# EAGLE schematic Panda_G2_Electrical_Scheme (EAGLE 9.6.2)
AUTHOR: Andrea Maroso; TITLE: Electrical Scheme

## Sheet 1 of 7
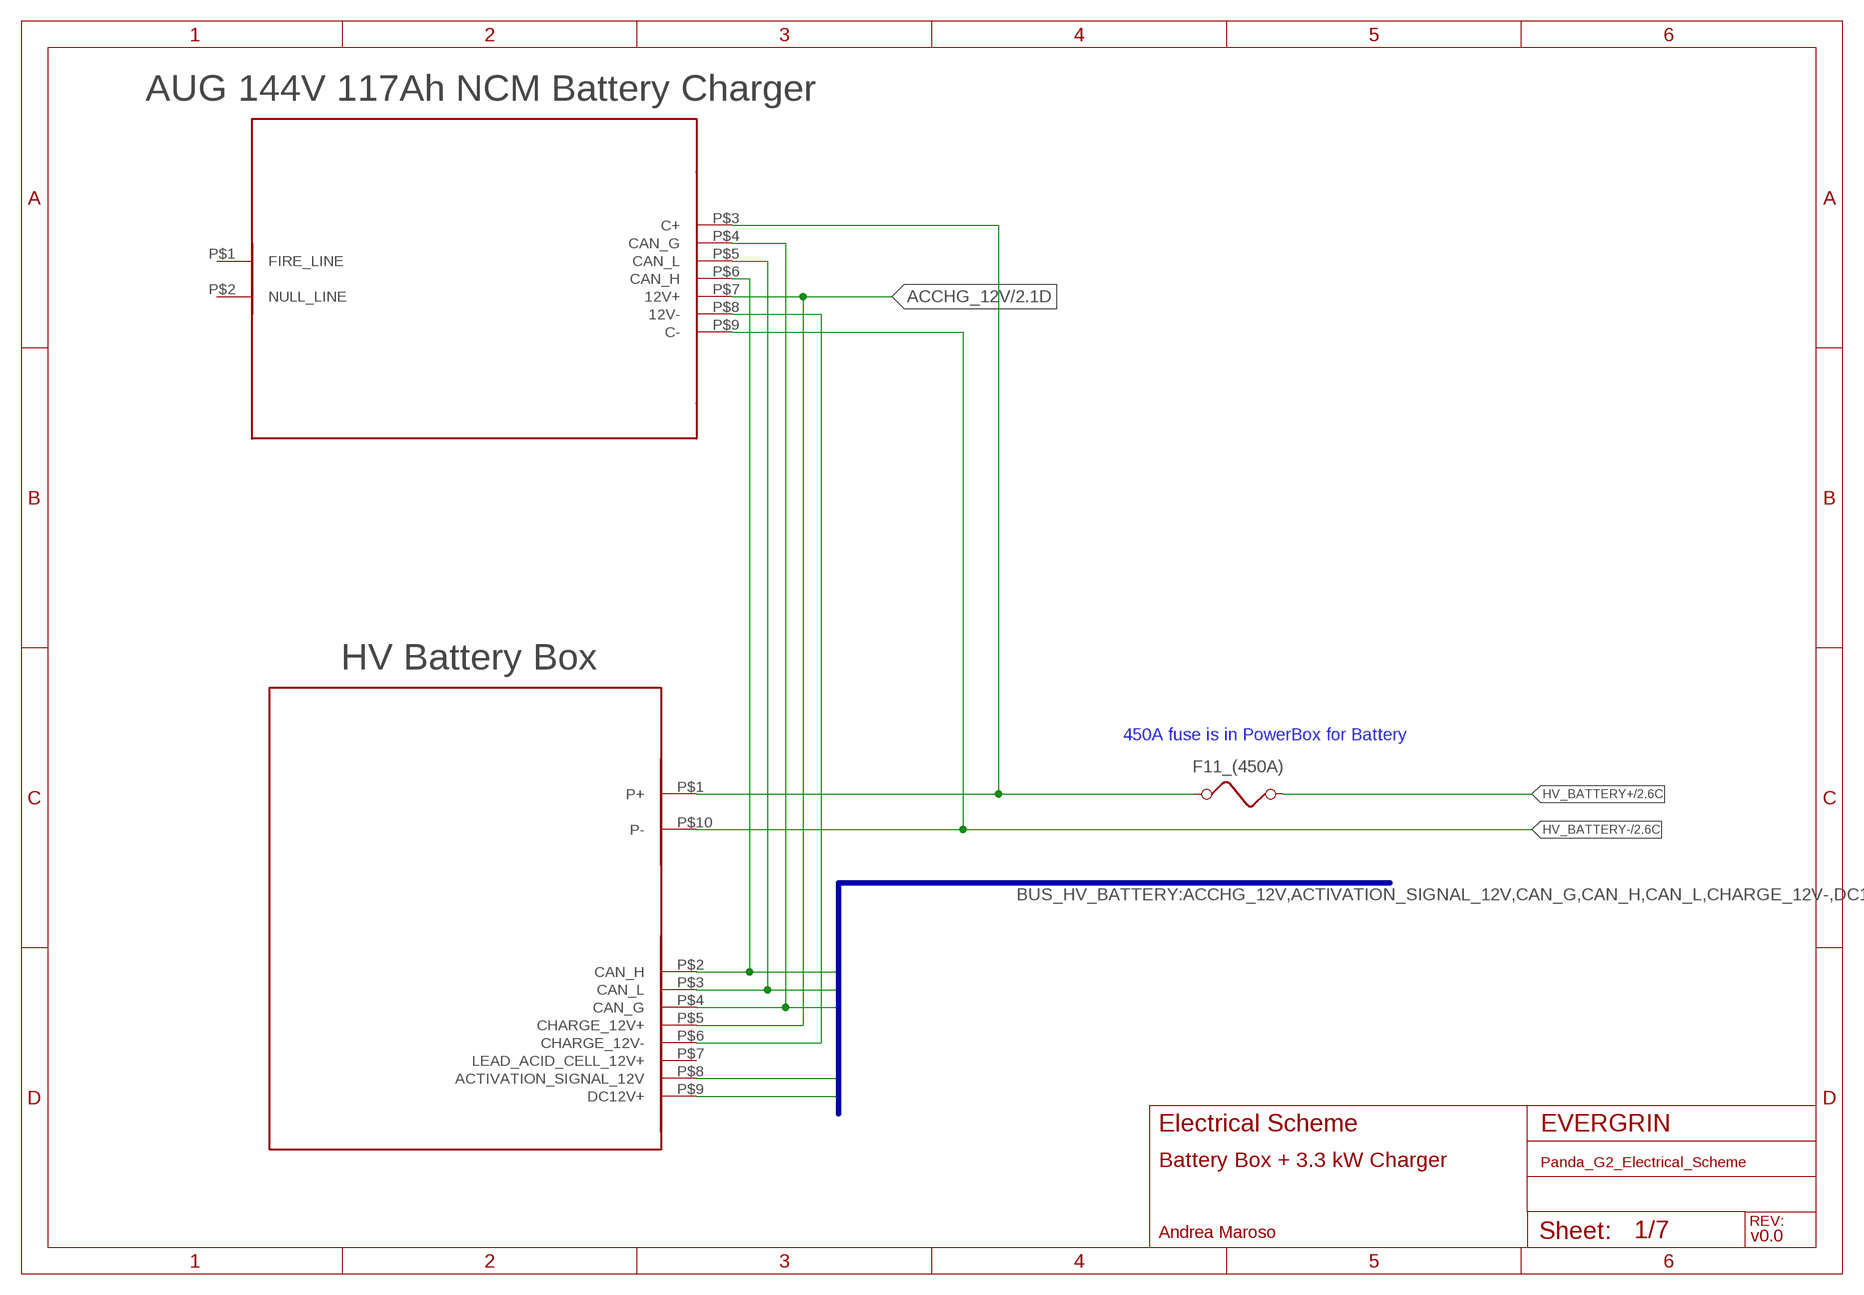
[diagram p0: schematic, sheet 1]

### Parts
F11_(450A)  FUSE  [FUSE]
U$1  HV_BATTERY_BOX  [HV_BATTERY_BOX]
U$2  1.8KW_BATTERY_CHARGER  [1.8KW_BATTERY_CHARGER]

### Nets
ACCHG_12V: U$1.P$5(CHARGE_12V+) U$2.P$7(12V+) ; also sheet 2,6
ACTIVATION_SIGNAL_12V: U$1.P$8(ACTIVATION_SIGNAL_12V) ; also sheet 6
CAN_G: U$1.P$4(CAN_G) U$2.P$4(CAN_G) ; also sheet 6
CAN_H: U$1.P$2(CAN_H) U$2.P$6(CAN_H) ; also sheet 2,6
CAN_L: U$1.P$3(CAN_L) U$2.P$5(CAN_L) ; also sheet 2,6
DC12V+: U$1.P$9(DC12V+) ; also sheet 6
HV_BATTERY+: F11_(450A).1 U$1.P$1(P+) U$2.P$3(C+) ; also sheet 2,4
HV_BATTERY+/2.6C: F11_(450A).2
HV_BATTERY-: U$1.P$10(P-) U$2.P$9(C-) ; also sheet 2,4
N$28: U$1.P$6(CHARGE_12V-) U$2.P$8(12V-)
Unconnected: U$1.P$7(LEAD_ACID_CELL_12V+) U$2.P$1(FIRE_LINE) U$2.P$2(NULL_LINE)

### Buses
BUS_HV_BATTERY:ACCHG_12V,ACTIVATION_SIGNAL_12V,CAN_G,CAN_H,CAN_L,CHARGE_12V-,DC12V+

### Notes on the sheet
- 450A fuse is in PowerBox for Battery
- Battery Box + 3.3 kW Charger
- v0.0

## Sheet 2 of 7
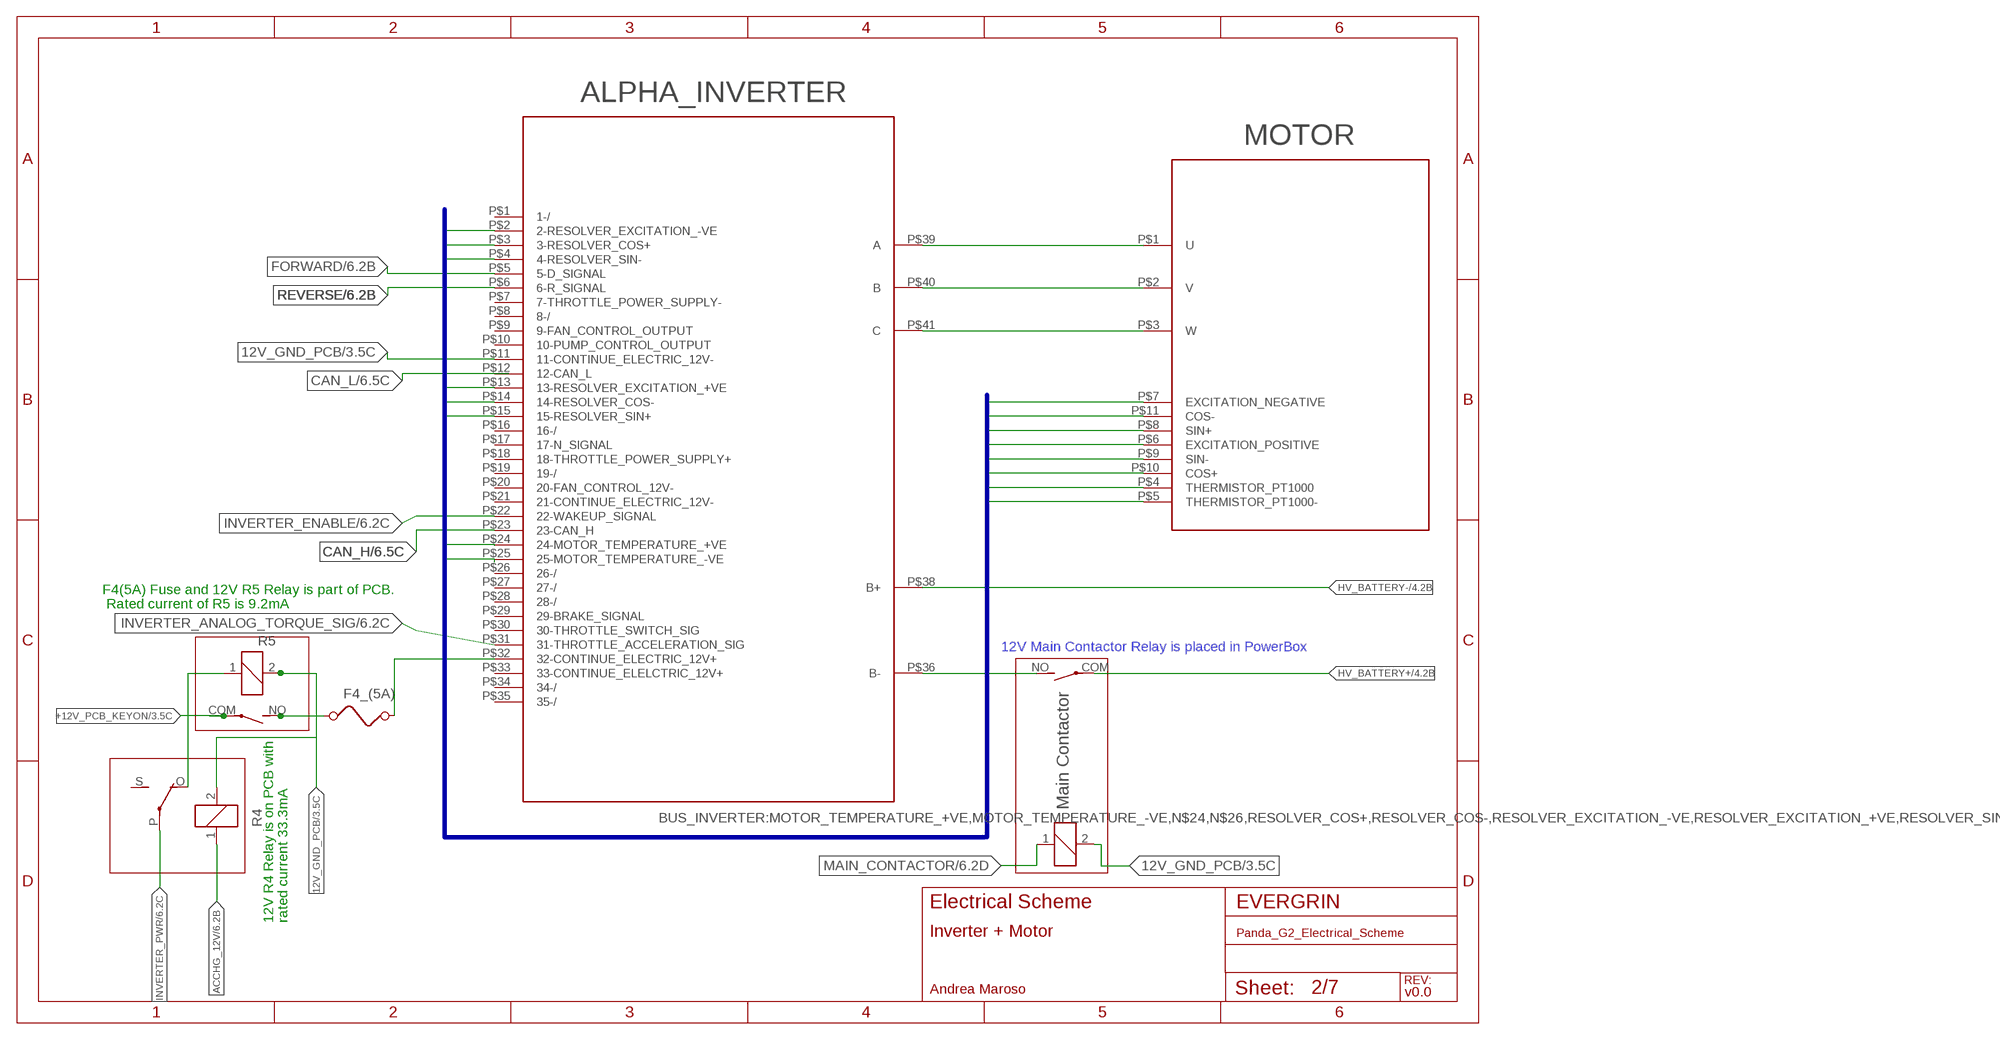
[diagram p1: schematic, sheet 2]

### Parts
F4_(5A)  FUSE  [FUSE]
K1  G5L  [G5LE]
MAIN_CONTACTOR  APF30212A  [APF30212A]
R5  APF30212A  [APF30212A]
U$3  INVERTER  [INVERTER]
U$4  MOTOR  [MOTOR]

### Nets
12V_GND_PCB: K1.2 MAIN_CONTACTOR.2 R5.2 U$3.P$11(11-CONTINUE_ELECTRIC_12V-) ; also sheet 3,4,5,6,7
+12V_PCB_KEYON: R5.COM(2:P) ; also sheet 3,5,7
ACCHG_12V: K1.1 ; also sheet 1,6
CAN_H: U$3.P$23(23-CAN_H) ; also sheet 1,6
CAN_L: U$3.P$12(12-CAN_L) ; also sheet 1,6
FORWARD: U$3.P$5(5-D_SIGNAL) ; also sheet 6
HV_BATTERY+: MAIN_CONTACTOR.COM(2:P) ; also sheet 1,4
HV_BATTERY-: U$3.P$38(B+) ; also sheet 1,4
INVERTER_ANALOG_TORQUE_SIG: U$3.P$31(31-THROTTLE_ACCELERATION_SIG) ; also sheet 6
INVERTER_ENABLE: U$3.P$22(22-WAKEUP_SIGNAL) ; also sheet 6
INVERTER_PWR: K1.P(2:P) ; also sheet 6
MAIN_CONTACTOR: MAIN_CONTACTOR.1 ; also sheet 6
N$1: F4_(5A).2 U$3.P$32(32-CONTINUE_ELECTRIC_12V+)
N$2: U$3.P$39(A) U$4.P$1(U)
N$3: U$3.P$40(B) U$4.P$2(V)
N$4: U$3.P$41(C) U$4.P$3(W)
N$5: MAIN_CONTACTOR.NO(2:S) U$3.P$36(B-)
N$23: F4_(5A).1 R5.NO(2:S)
N$24: U$3.P$24(24-MOTOR_TEMPERATURE_+VE) U$4.P$4(THERMISTOR_PT1000)
N$25: K1.O(2:O) R5.1
N$26: U$3.P$25(25-MOTOR_TEMPERATURE_-VE) U$4.P$5(THERMISTOR_PT1000-)
RESOLVER_COS+: U$3.P$3(3-RESOLVER_COS+) U$4.P$10(COS+)
RESOLVER_COS-: U$3.P$14(14-RESOLVER_COS-) U$4.P$11(COS-)
RESOLVER_EXCITATION_+VE: U$3.P$13(13-RESOLVER_EXCITATION_+VE) U$4.P$6(EXCITATION_POSITIVE)
RESOLVER_EXCITATION_-VE: U$3.P$2(2-RESOLVER_EXCITATION_-VE) U$4.P$7(EXCITATION_NEGATIVE)
RESOLVER_SIN+: U$3.P$15(15-RESOLVER_SIN+) U$4.P$8(SIN+)
RESOLVER_SIN-: U$3.P$4(4-RESOLVER_SIN-) U$4.P$9(SIN-)
REVERSE: U$3.P$6(6-R_SIGNAL) ; also sheet 6
Unconnected: K1.S(2:S) U$3.P$1(1-/) U$3.P$7(7-THROTTLE_POWER_SUPPLY-) U$3.P$8(8-/) U$3.P$9(9-FAN_CONTROL_OUTPUT) U$3.P$10(10-PUMP_CONTROL_OUTPUT) U$3.P$16(16-/) U$3.P$17(17-N_SIGNAL) U$3.P$18(18-THROTTLE_POWER_SUPPLY+) U$3.P$19(19-/) U$3.P$20(20-FAN_CONTROL_12V-) U$3.P$21(21-CONTINUE_ELECTRIC_12V-) U$3.P$26(26-/) U$3.P$27(27-/) U$3.P$28(28-/) U$3.P$29(29-BRAKE_SIGNAL) U$3.P$30(30-THROTTLE_SWITCH_SIG) U$3.P$33(33-CONTINUE_ELELCTRIC_12V+) U$3.P$34(34-/) U$3.P$35(35-/)

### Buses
BUS_INVERTER:MOTOR_TEMPERATURE_+VE,MOTOR_TEMPERATURE_-VE,N$24,N$26,RESOLVER_COS+,RESOLVER_COS-,RESOLVER_EXCITATION_-VE,RESOLVER_EXCITATION_+VE,RESOLVER_SIN-,RESOLVER_SIN+

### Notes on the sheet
- F4(5A) Fuse and 12V R5 Relay is part of PCB.
- Rated current of R5 is 9.2mA
- 12V Main Contactor Relay is placed in PowerBox
- Main Contactor
- R4
- 12V R4 Relay is on PCB with | rated current 33.3mA
- Inverter + Motor
- v0.0

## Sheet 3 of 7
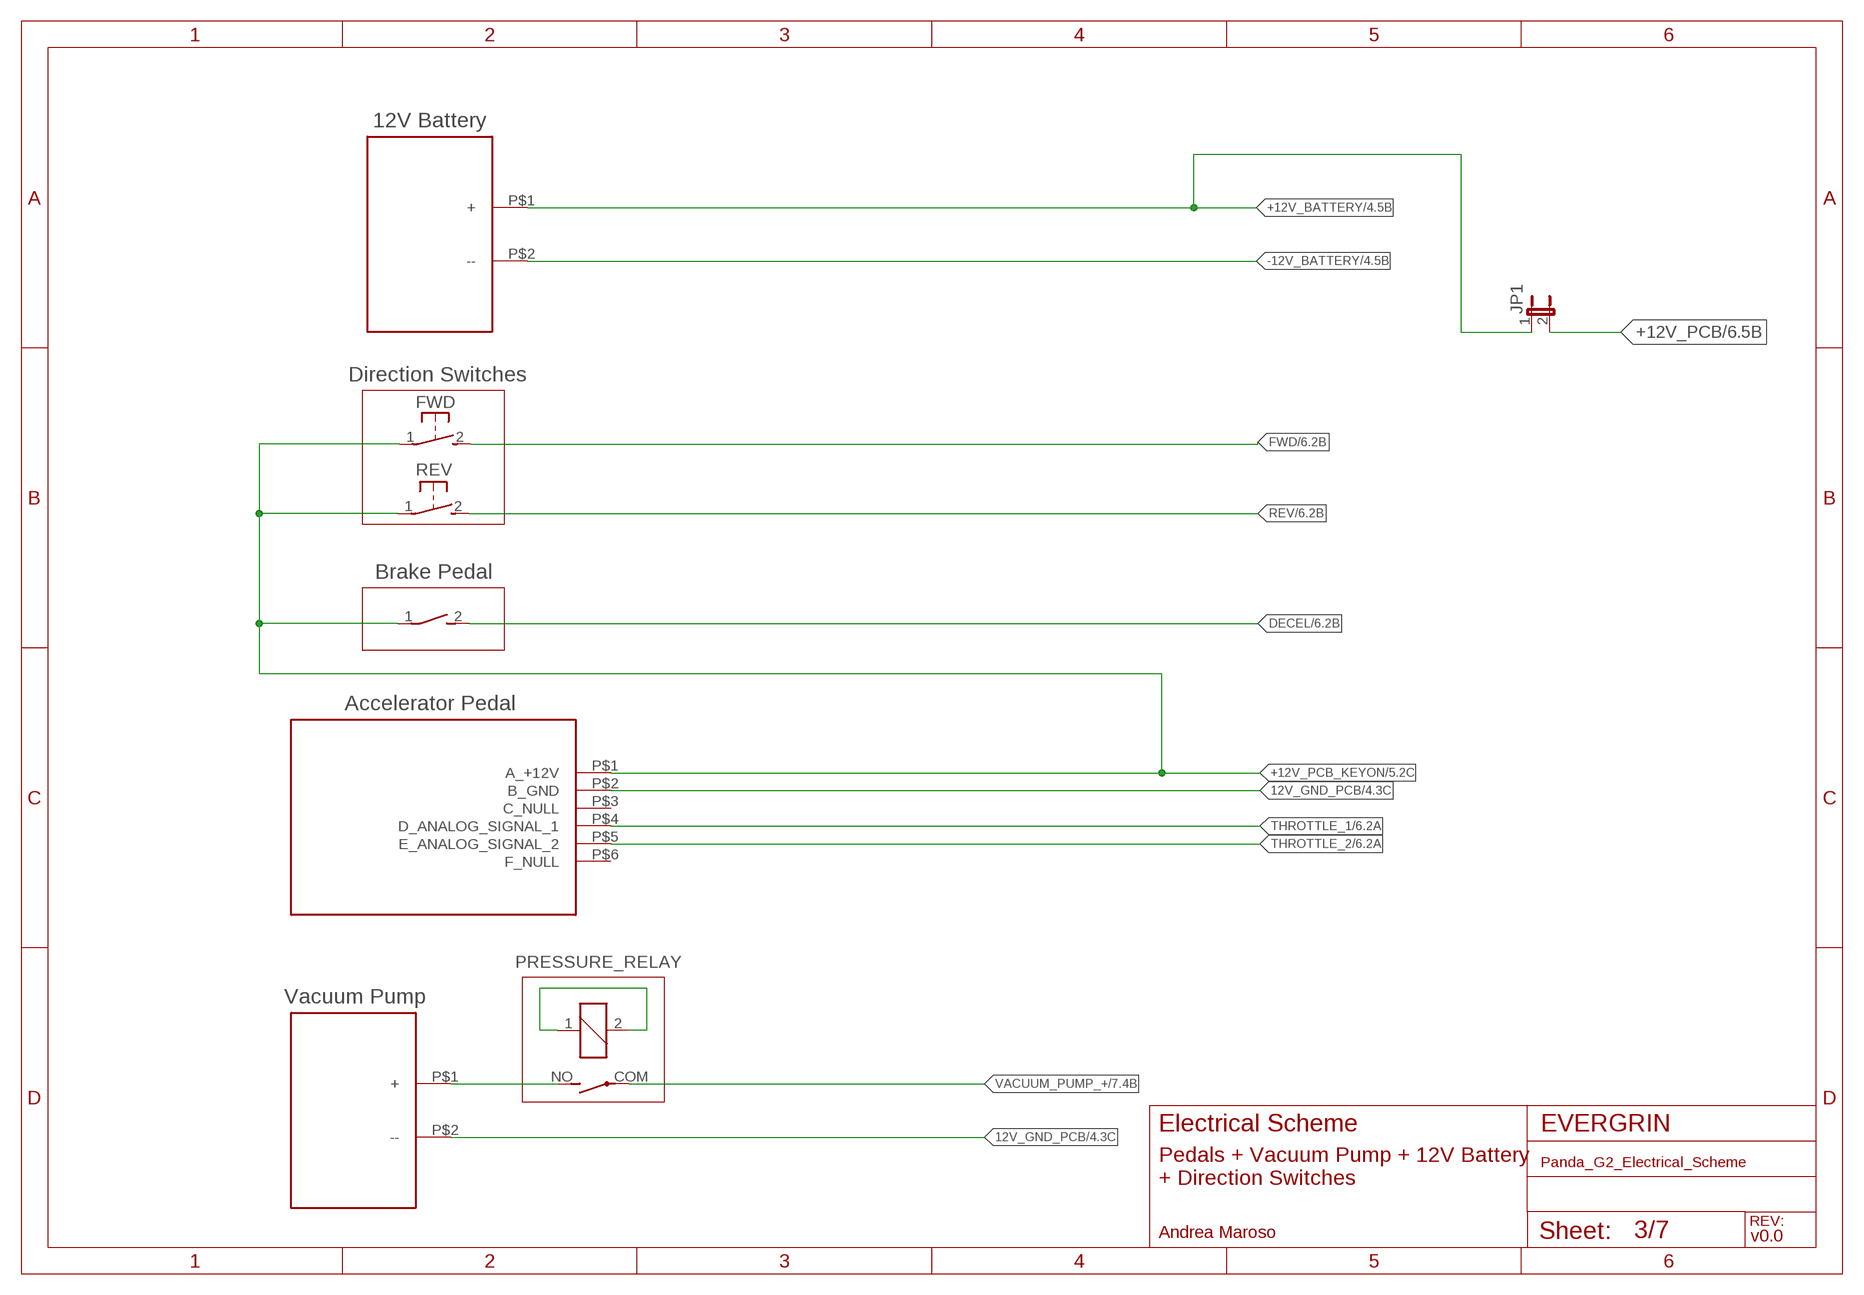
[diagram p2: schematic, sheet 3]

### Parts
JP1  JP1E  [JP1]
PRESSURE_RELAY  APF30212A  [APF30212A]
S1  31-XX  [B3F-31XX]
S2  31-XX  [B3F-31XX]
S4  DS01E  [DS-01]
U$5  12V_BATTERY  [12V_BATTERY]
U$6  ACC_PEDAL  [ACC_PEDAL]
U$7  VACUUM_PUMP  [VACUUM_PUMP]

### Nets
12V_GND_PCB: U$6.P$2(B_GND) U$7.P$2(--) ; also sheet 2,4,5,6,7
+12V_BATTERY: JP1.1 U$5.P$1(+) ; also sheet 4,6
+12V_PCB: JP1.2 ; also sheet 6,7
+12V_PCB_KEYON: S1.1(P) S2.1(P) S4.1 U$6.P$1(A_+12V) ; also sheet 2,5,7
-12V_BATTERY: U$5.P$2(--) ; also sheet 4
DECEL: S4.2 ; also sheet 6
FWD: S1.2(S) ; also sheet 6
N$7: PRESSURE_RELAY.1 PRESSURE_RELAY.2
REV: S2.2(S) ; also sheet 6
THROTTLE_1: U$6.P$4(D_ANALOG_SIGNAL_1) ; also sheet 6
THROTTLE_2: U$6.P$5(E_ANALOG_SIGNAL_2) ; also sheet 6
VACUUM_PUMP_+: PRESSURE_RELAY.COM(2:P) PRESSURE_RELAY.NO(2:S) U$7.P$1(+) ; also sheet 7
Unconnected: U$6.P$3(C_NULL) U$6.P$6(F_NULL)

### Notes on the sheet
- Direction Switches
- FWD
- REV
- Brake Pedal
- Pedals + Vacuum Pump + 12V Battery
  + Direction Switches
- v0.0

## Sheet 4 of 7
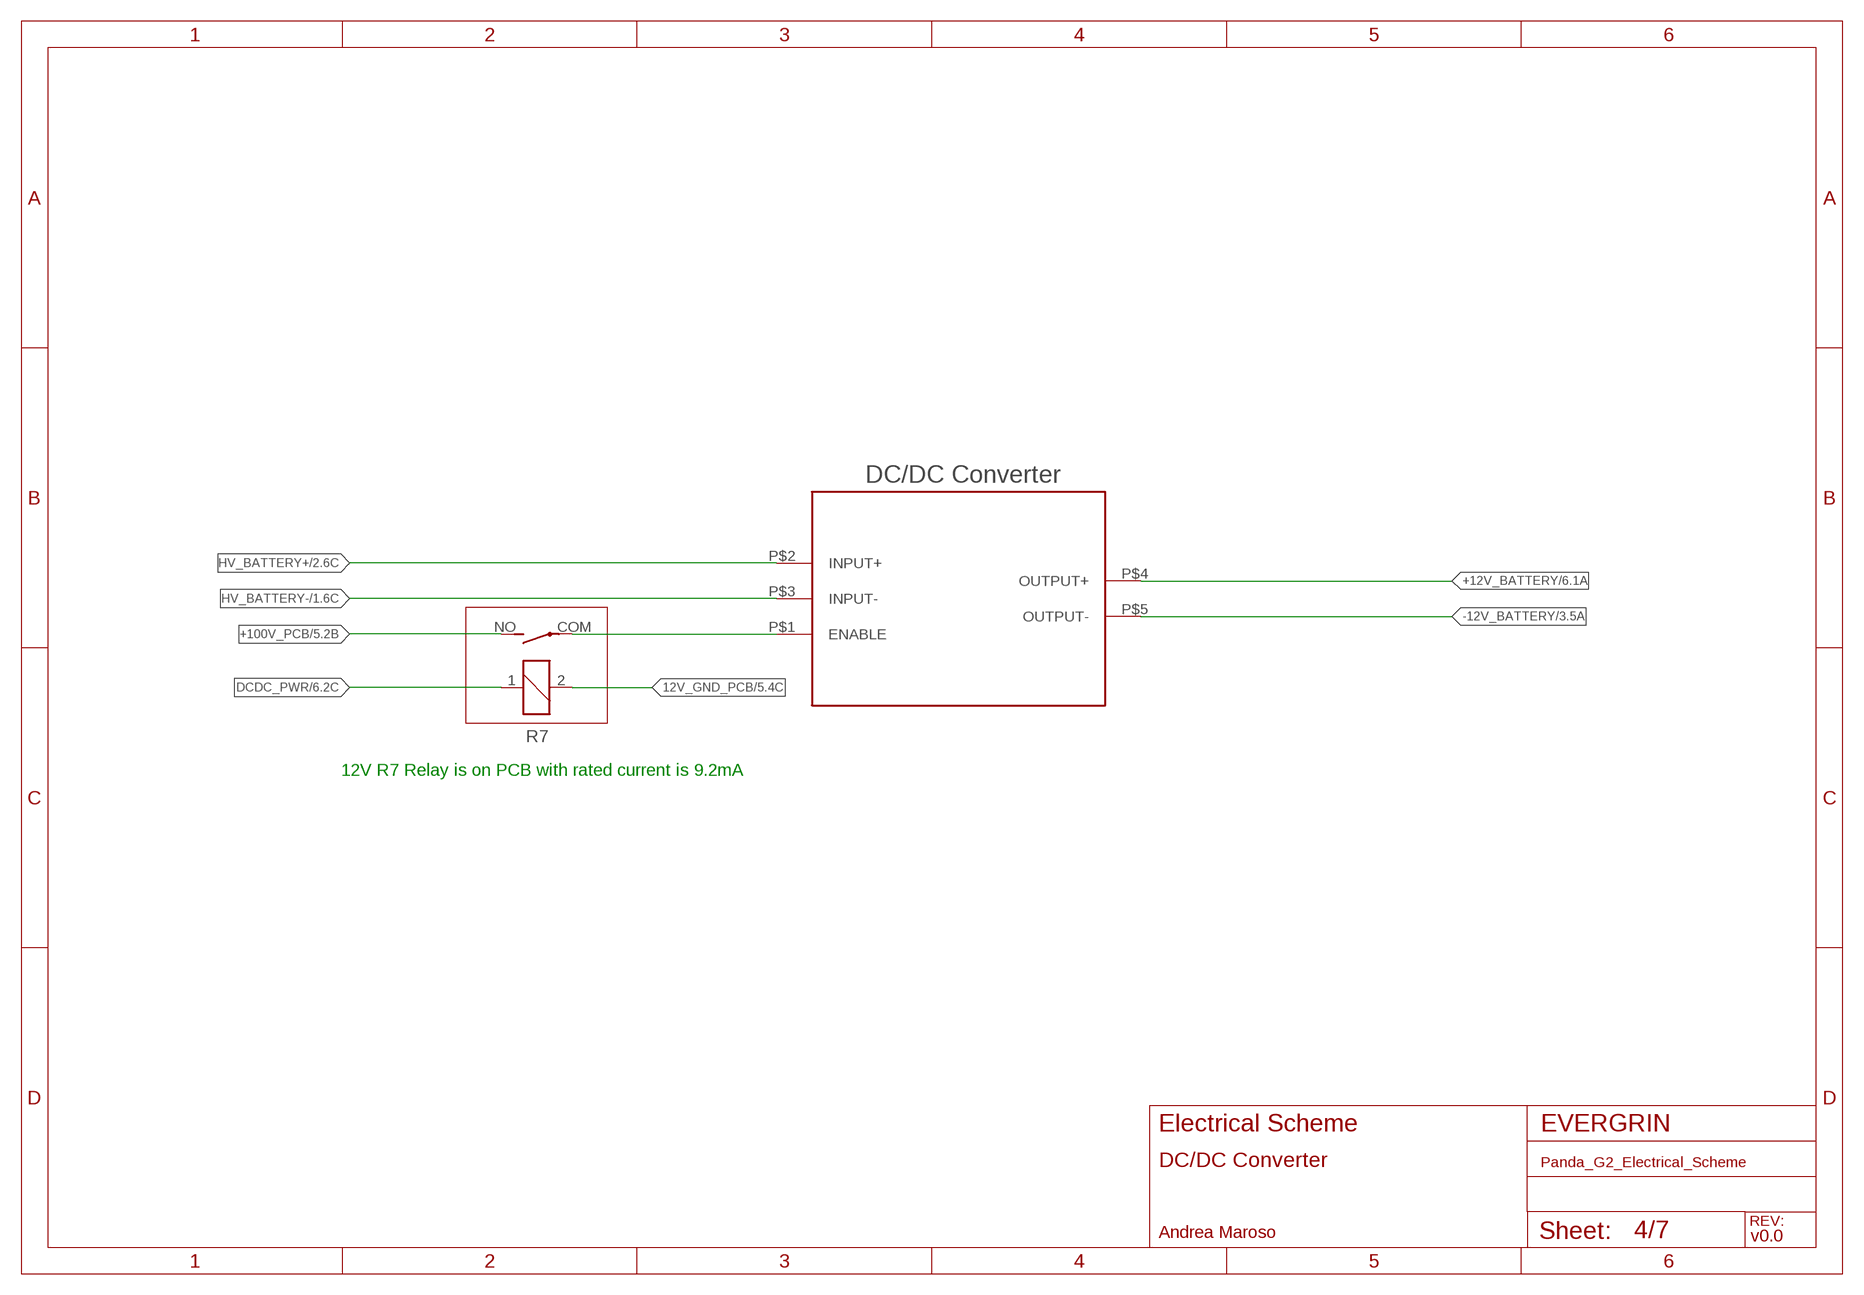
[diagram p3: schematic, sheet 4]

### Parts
R7  APF30212A  [APF30212A]
U$8  DC/DC  [DC/DC]

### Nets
12V_GND_PCB: R7.2 ; also sheet 2,3,5,6,7
+12V_BATTERY: U$8.P$4(OUTPUT+) ; also sheet 3,6
+100V_PCB: R7.NO(2:S) ; also sheet 5
-12V_BATTERY: U$8.P$5(OUTPUT-) ; also sheet 3
DCDC_PWR: R7.1 ; also sheet 6
HV_BATTERY+: U$8.P$2(INPUT+) ; also sheet 1,2
HV_BATTERY-: U$8.P$3(INPUT-) ; also sheet 1,2
N$6: R7.COM(2:P) U$8.P$1(ENABLE)

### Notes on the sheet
- 12V R7 Relay is on PCB with rated current is 9.2mA
- DC/DC Converter
- v0.0

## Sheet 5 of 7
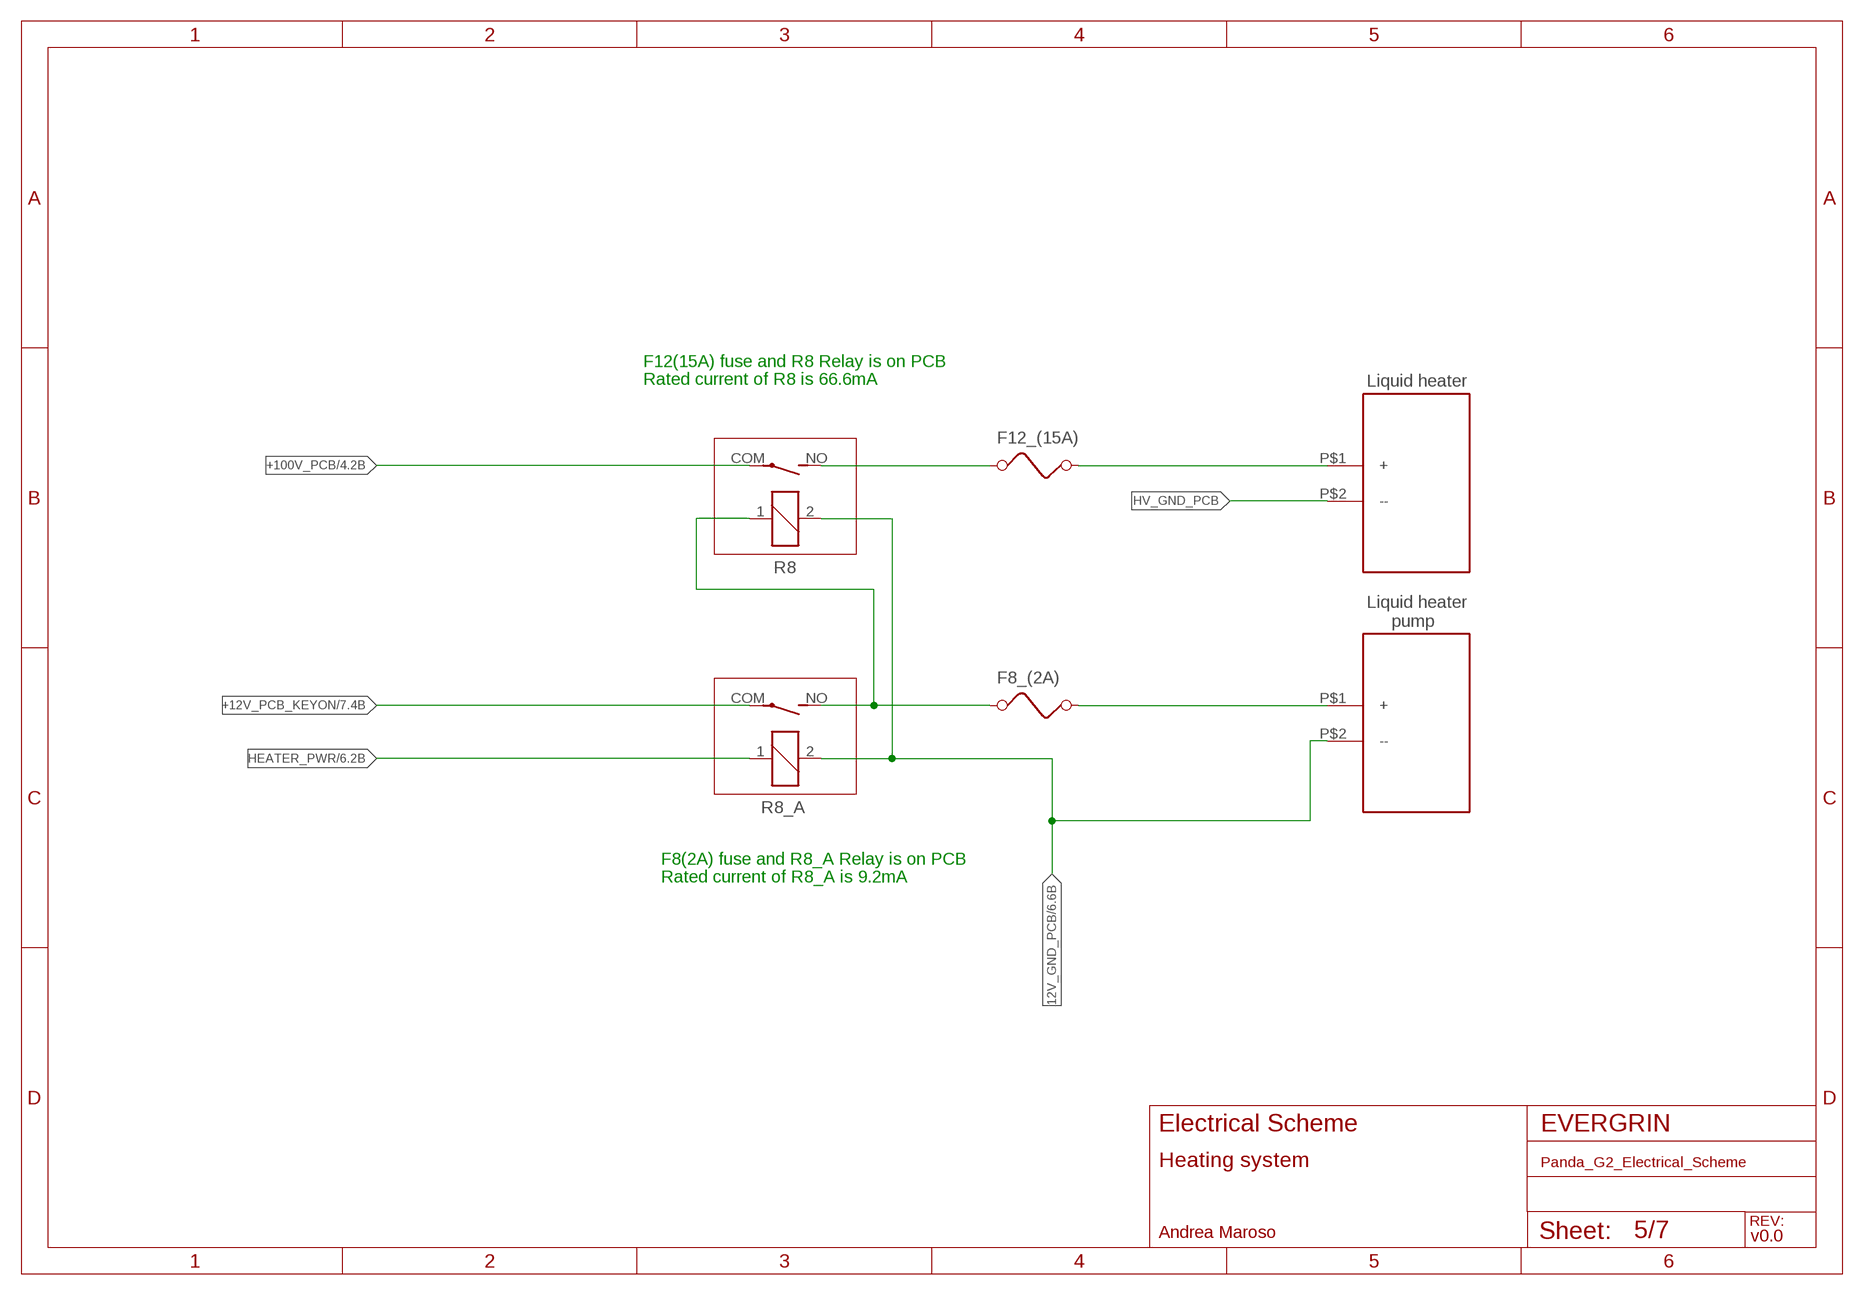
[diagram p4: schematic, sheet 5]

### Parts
F8_(2A)  FUSE  [FUSE]
F12_(15A)  FUSE  [FUSE]
R8  APF30212A  [APF30212A]
R8_A  APF30212A  [APF30212A]
U$9  LIQUID_HEATER  [LIQUID_HEATER]
U$10  LIQUID_HEATER_PUMP  [LIQUID_HEATER_PUMP]

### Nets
12V_GND_PCB: R8.2 R8_A.2 U$10.P$2(--) ; also sheet 2,3,4,6,7
+12V_PCB_KEYON: R8_A.COM(2:P) ; also sheet 2,3,7
+100V_PCB: R8.COM(2:P) ; also sheet 4
HEATER_PWR: R8_A.1 ; also sheet 6
HV_GND_PCB: U$9.P$2(--)
N$8: F12_(15A).1 R8.NO(2:S)
N$9: F12_(15A).2 U$9.P$1(+)
N$11: F8_(2A).1 R8.1 R8_A.NO(2:S)
N$12: F8_(2A).2 U$10.P$1(+)

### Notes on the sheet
- F12(15A) fuse and R8 Relay is on PCB
- Rated current of R8 is 66.6mA
- F8(2A) fuse and R8_A Relay is on PCB
- Rated current of R8_A is 9.2mA
- Heating system
- v0.0

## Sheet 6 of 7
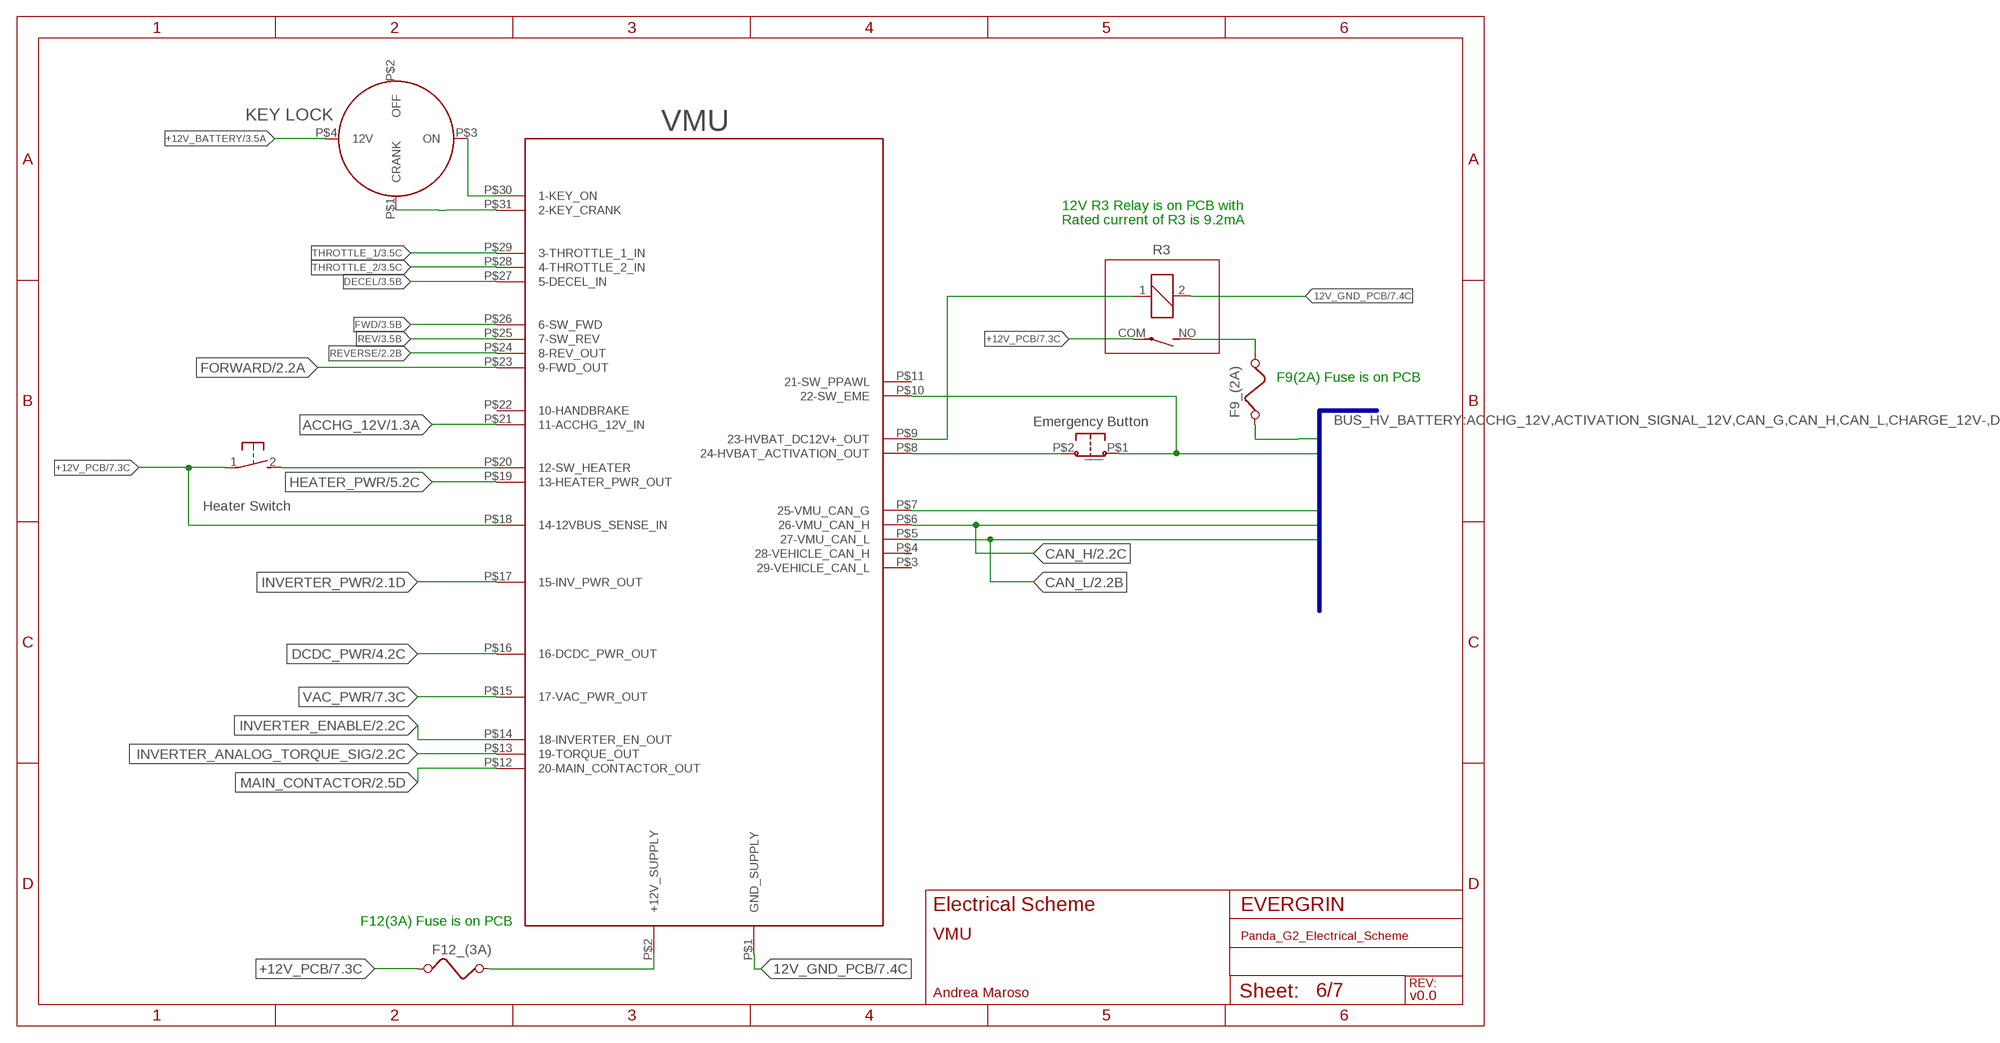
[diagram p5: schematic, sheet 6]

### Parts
F9_(2A)  FUSE  [FUSE]
F12_(3A)  FUSE  [FUSE]
R3  APF30212A  [APF30212A]
S5  31-XX  [B3F-31XX]
U$11  VMU  [VMU]
U$12  IGNITION_LOCK  [IGNITION_LOCK]
U$13  EMERGENCY_BUTTON  [EMERGENCY_BUTTON]

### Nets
12V_GND_PCB: R3.2 U$11.P$1(GND_SUPPLY) ; also sheet 2,3,4,5,7
+12V_BATTERY: U$12.P$4(12V) ; also sheet 3,4
+12V_PCB: F12_(3A).1 R3.COM(2:P) S5.1(P) U$11.P$18(14-12VBUS_SENSE_IN) ; also sheet 3,7
ACCHG_12V: U$11.P$21(11-ACCHG_12V_IN) ; also sheet 1,2
ACTIVATION_SIGNAL_12V: U$11.P$10(22-SW_EME) U$13.P$1(_) ; also sheet 1
CAN_G: U$11.P$7(25-VMU_CAN_G) ; also sheet 1
CAN_H: U$11.P$4(28-VEHICLE_CAN_H) U$11.P$6(26-VMU_CAN_H) ; also sheet 1,2
CAN_L: U$11.P$5(27-VMU_CAN_L) ; also sheet 1,2
DC12V+: F9_(2A).2 ; also sheet 1
DCDC_PWR: U$11.P$16(16-DCDC_PWR_OUT) ; also sheet 4
DECEL: U$11.P$27(5-DECEL_IN) ; also sheet 3
FORWARD: U$11.P$23(9-FWD_OUT) ; also sheet 2
FWD: U$11.P$26(6-SW_FWD) ; also sheet 3
HEATER_PWR: U$11.P$19(13-HEATER_PWR_OUT) ; also sheet 5
INVERTER_ANALOG_TORQUE_SIG: U$11.P$13(19-TORQUE_OUT) ; also sheet 2
INVERTER_ENABLE: U$11.P$14(18-INVERTER_EN_OUT) ; also sheet 2
INVERTER_PWR: U$11.P$17(15-INV_PWR_OUT) ; also sheet 2
KEY_CRANK: U$11.P$31(2-KEY_CRANK) U$12.P$1(CRANK)
KEY_ON: U$11.P$30(1-KEY_ON) U$12.P$3(ON) ; also sheet 7
MAIN_CONTACTOR: U$11.P$12(20-MAIN_CONTACTOR_OUT) ; also sheet 2
N$13: S5.2(S) U$11.P$20(12-SW_HEATER)
N$14: F12_(3A).2 U$11.P$2(+12V_SUPPLY)
N$16: F9_(2A).1 R3.NO(2:S)
N$17: U$11.P$8(24-HVBAT_ACTIVATION_OUT) U$13.P$2(__)
N$29: R3.1 U$11.P$9(23-HVBAT_DC12V+_OUT)
REV: U$11.P$25(7-SW_REV) ; also sheet 3
REVERSE: U$11.P$24(8-REV_OUT) ; also sheet 2
THROTTLE_1: U$11.P$29(3-THROTTLE_1_IN) ; also sheet 3
THROTTLE_2: U$11.P$28(4-THROTTLE_2_IN) ; also sheet 3
VAC_PWR: U$11.P$15(17-VAC_PWR_OUT) ; also sheet 7
Unconnected: U$11.P$3(29-VEHICLE_CAN_L) U$11.P$11(21-SW_PPAWL) U$11.P$22(10-HANDBRAKE) U$12.P$2(OFF)

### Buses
BUS_HV_BATTERY:ACCHG_12V,ACTIVATION_SIGNAL_12V,CAN_G,CAN_H,CAN_L,CHARGE_12V-,DC12V+

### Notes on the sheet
- 12V R3 Relay is on PCB with
- Rated current of R3 is 9.2mA
- F9(2A) Fuse is on PCB
- Heater Switch
- F12(3A) Fuse is on PCB
- VMU
- v0.0

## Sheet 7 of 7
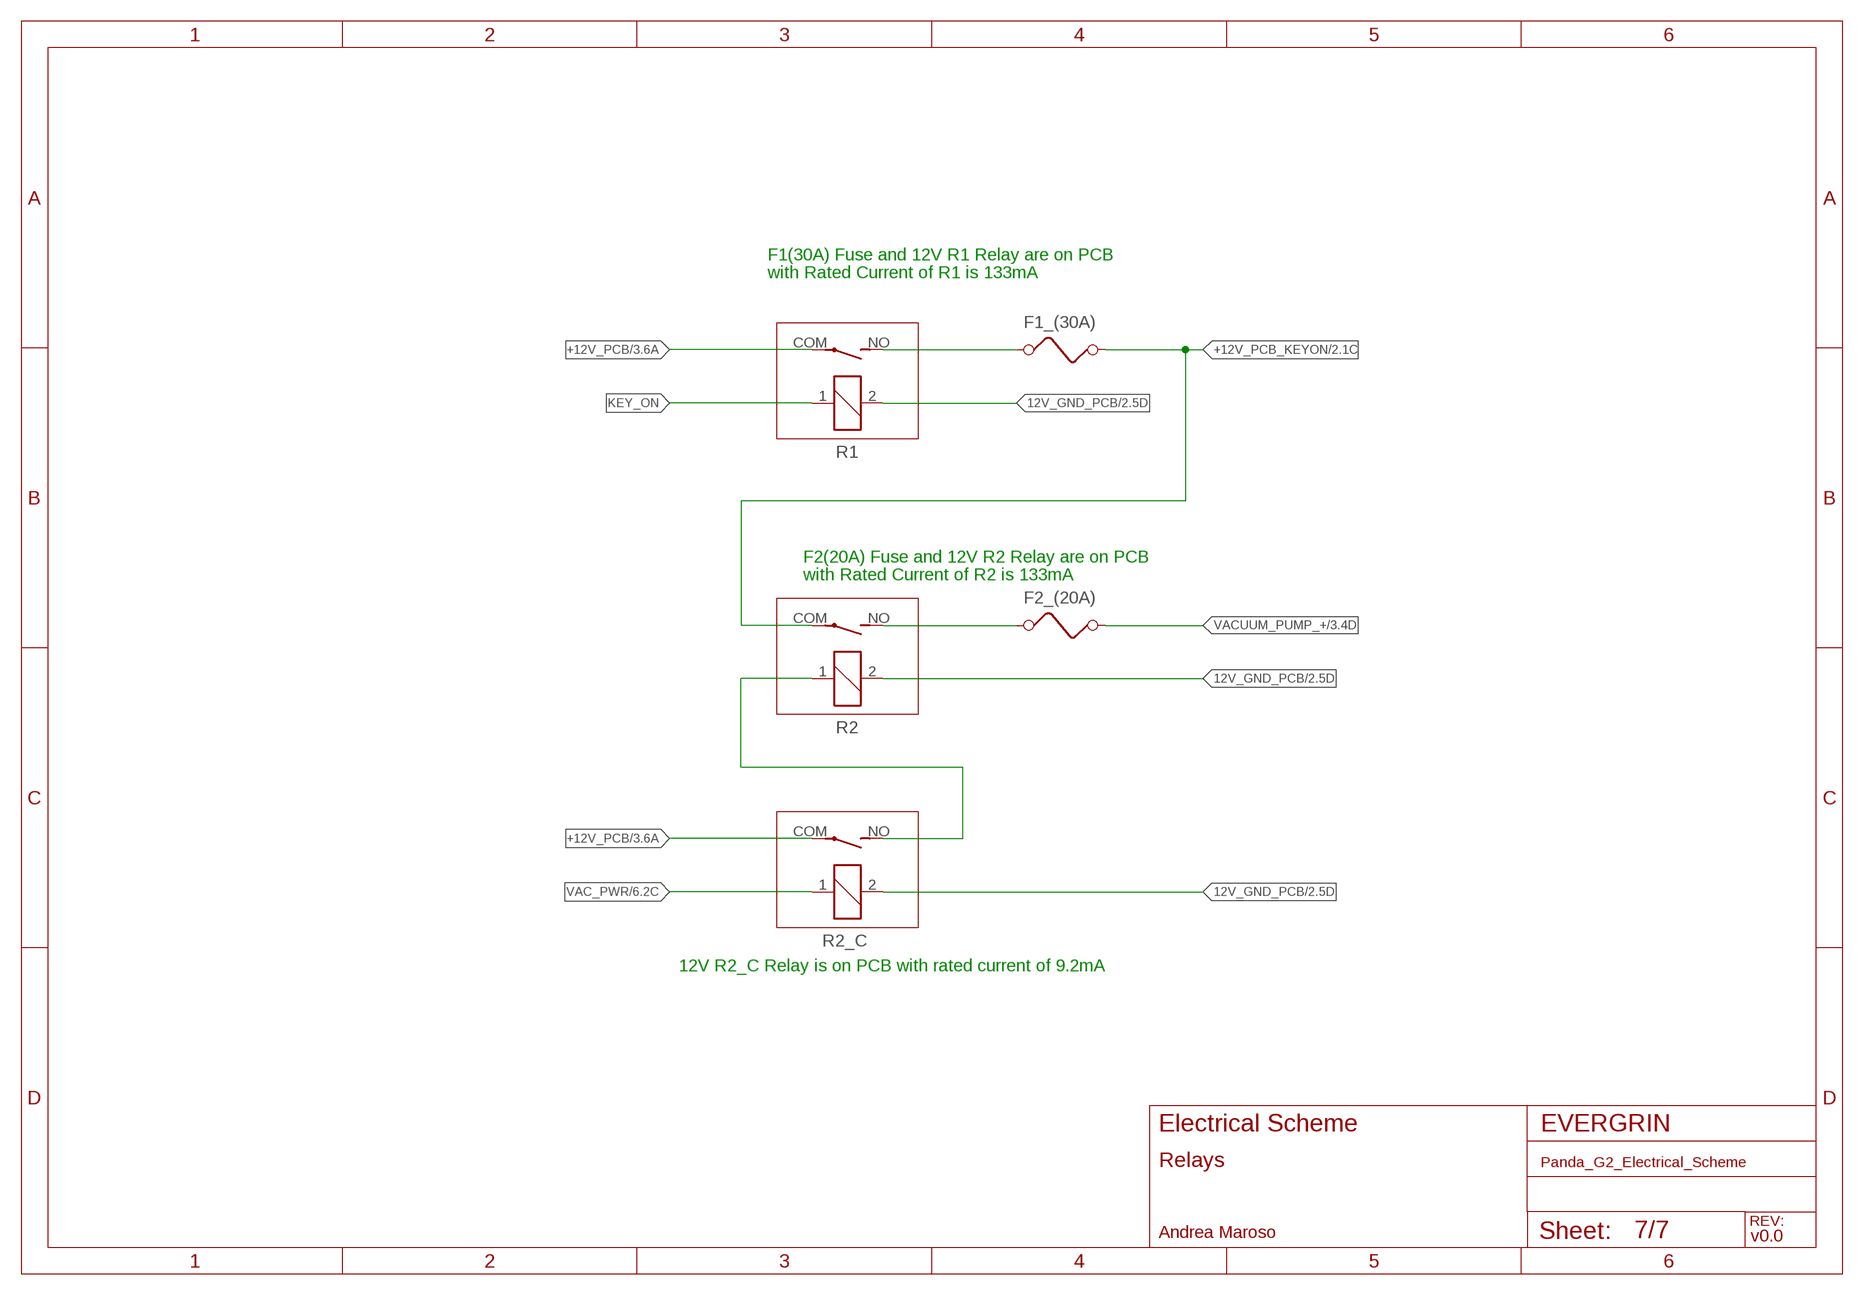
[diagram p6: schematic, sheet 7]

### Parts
F1_(30A)  FUSE  [FUSE]
F2_(20A)  FUSE  [FUSE]
R1  APF30212A  [APF30212A]
R2  APF30212A  [APF30212A]
R2_C  APF30212A  [APF30212A]

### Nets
12V_GND_PCB: R1.2 R2.2 R2_C.2 ; also sheet 2,3,4,5,6
+12V_PCB: R1.COM(2:P) R2_C.COM(2:P) ; also sheet 3,6
+12V_PCB_KEYON: F1_(30A).2 R2.COM(2:P) ; also sheet 2,3,5
KEY_ON: R1.1 ; also sheet 6
N$10: F2_(20A).1 R2.NO(2:S)
N$20: F1_(30A).1 R1.NO(2:S)
N$22: R2.1 R2_C.NO(2:S)
VAC_PWR: R2_C.1 ; also sheet 6
VACUUM_PUMP_+: F2_(20A).2 ; also sheet 3

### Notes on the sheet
- F1(30A) Fuse and 12V R1 Relay are on PCB
- with Rated Current of R1 is 133mA
- F2(20A) Fuse and 12V R2 Relay are on PCB
- with Rated Current of R2 is 133mA
- 12V R2_C Relay is on PCB with rated current of 9.2mA
- Relays
- v0.0

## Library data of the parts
F1_(30A) F2_(20A) F4_(5A) F8_(2A) F9_(2A) F11_(450A) F12_(3A) F12_(15A) = special:FUSE: FUSE
JP1 = jumper:JP1E: JUMPER
K1 = relay:G5L: RELAY 1 x switch, 10 A/120 V AC, 8 A/30 V ADC, Omron; OC_FARNELL: unknown; OC_NEWARK: unknown
MAIN_CONTACTOR PRESSURE_RELAY R1 R2 R2_C R3 R5 R7 R8 R8_A = relay:APF30212A: Compliant with European standards 1a/1c 6A Slim power relays Source: Data sheet; OC_FARNELL: unknown
S1 S2 S5 = switch-omron:31-XX: OMRON SWITCH; MPN: B3F-3100; OC_FARNELL: 959704; OC_NEWARK: 36M3582
S4 = switch-dil:DS01E: DIL/CODE SWITCH; OC_FARNELL: unknown; OC_NEWARK: unknown
U$1 = EVERGRIN_Panda_G2:HV_BATTERY_BOX: HV battery box
U$2 = EVERGRIN_Panda_G2:1.8KW_BATTERY_CHARGER: 1.8 kW battery charger
U$3 = EVERGRIN_Panda_G2:INVERTER: Inverter
U$4 = EVERGRIN_Panda_G2:MOTOR: Motor
U$5 = EVERGRIN_Panda_G2:12V_BATTERY: 12 V battery
U$6 = EVERGRIN_Panda_G2:ACC_PEDAL: Accelerator pedal
U$7 = EVERGRIN_Panda_G2:VACUUM_PUMP
U$8 = EVERGRIN_Panda_G2:DC/DC
U$9 = EVERGRIN_Panda_G2:LIQUID_HEATER: Liquid Heater
U$10 = EVERGRIN_Panda_G2:LIQUID_HEATER_PUMP: Liquid Heater Pump
U$11 = EVERGRIN_Panda_G2:VMU
U$12 = EVERGRIN_Panda_G2:IGNITION_LOCK
U$13 = EVERGRIN_Panda_G2:EMERGENCY_BUTTON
